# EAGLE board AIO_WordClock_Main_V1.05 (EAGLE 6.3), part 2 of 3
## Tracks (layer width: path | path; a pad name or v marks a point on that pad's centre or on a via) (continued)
+3V3  (via drill 0.5, 0.6) (continued)
  Bottom 0.406: 138.15,300.52 137.36,299.73 C104.1 136.66,299.65 C103.1 | 138.15,238.52 137.36,237.73 C204.1 136.66,237.66 C203.1 | 138.15,176.52 137.36,175.73 C304.1 136.66,175.66 C303.1 | 138.15,114.52 137.36,113.73 C404.1 136.66,113.66 C403.1 | 138.15,52.52 137.36,51.73 C504.1 136.66,51.66 C503.1 | U703.2 210.87,51.26 C704.1 208.22,51.26 208,51.47 208,55.03 | 198.96,55.03 208,55.03 | 208,55.03 211.05,58.08 242.42,58.08 v245.34,61 | C710.1 217.38,41.74 U704.45 220.44,41.74 v220.57,41.87 | C712.1 217.38,33.74 U704.35 220.47,33.74 v220.57,33.85 | C709.1 225.87,28.76 226.53,29.41 U704.25 226.53,31.68 v226.42,31.79 | C708.1 236.47,32.94 U704.15 233.36,32.94 v233.28,32.88 | C711.1 224.12,47.69 U704.53 224.12,44.49 v224.18,44.49 | C713.1 230.53,47.69 U704.61 230.53,44.62 v230.66,44.49 | R705.1 264.66,69.75 v264.52,69.89 | R706.1 R707.1 162.45,23.7 v163.43,24.68 | J701.4 227.56,331.51 309.22,331.51 311.13,329.6 311.13,85
  Bottom 0.61: v136.65,295.82 C103.1 | C203.1 136.66,234.26 v136.12,233.72 | C303.1 136.66,172.53 v135.87,171.74 | C403.1 136.66,110.56 v135.87,109.77 | C503.1 136.66,48.45 v135.87,47.66 | R701.1 196.67,96.33 198.99,94.02 198.96,55.03 198.96,53.13 198.96,51.09 198.96,49.06 | 236.42,30.82 v235.16,30.82 | 236.42,30.82 C714.1 | 236.42,30.82 236.58,30.67 v236.58,24.68 | v285.73,21.76 285.73,46.14 290.43,50.84 290.43,56.94 | 290.43,56.94 290.43,81.32 291.69,82.59 308.71,82.59 311.13,85 | R703.1 290.51,57.03 290.43,56.94 | v300.84,21.76 301.09,21.76 303.12,19.72 303.12,10.2 J701A.4
  Bottom 1.016: v131.04,295.82 v131.04,233.72 v131.04,171.74 v131.04,109.77 v131.04,47.66 v131.04,24.68 | v198.96,24.68 198.96,49.06 | v225.02,17.82 J702.3
+3V3A  (via drill 0.5)
  Top 0.406: J603.10 179.17,14.01 J603.9 177.65,16.8 162.79,16.8 161.9,15.91 161.9,10.94 v165.2,7.63 165.21,7.52 U602.4
  Bottom 0.406: C609.1 165.34,7.39 v165.2,7.63
D+
  Top 0.254: U602.15 171.71,11.94 172.57,11.09 178.54,11.09 179.05,10.58 179.05,9.56 179.17,9.44 J602.3
D-
  Top 0.254: U602.16 171.06,11.83 172.31,10.58 178.28,10.58 178.54,10.33 178.54,9.56 178.37,9.4 J602.2
DCF77#  (via drill 0.5, 0.6)
  Top 0.254: v255.5,23.03 v283.06,23.03 v294.87,23.03
  Bottom 0.254: v255.5,23.03 255.5,33.43 249.59,39.34 U704.7 | J701.2 228.19,329.73 228.83,330.37 308.97,330.37 310.11,329.22 310.11,86.53 307.95,84.37 290.81,84.37 288.65,82.21 288.65,51.73 283.69,46.78 283.69,24.8 283.06,24.17 v283.06,23.03 | v294.87,23.03 301.47,23.03 303.76,20.74 303.76,10.96 307.57,7.15 307.57,5.75 J701A.2
DISP-A0
  Bottom 0.254: J702.2 226.29,19.47 232.12,25.31 U704.18
DISP-CLK
  Bottom 0.254: J702.7 219.94,16.68 228.96,25.69 228.96,28.79 228.12,29.62 U704.23
DISP-CS#
  Bottom 0.254: J702.5 222.48,17.44 230.53,25.48 U704.20
DISP-DIN
  Bottom 0.254: J702.6 221.21,17.06 229.72,25.57 U704.21
DISP-RESET#
  Bottom 0.254: J702.4 223.75,17.82 231.32,25.39 U704.19
GND  (via drill 0.5, 3)
  Top 0.406: U601.HS 286.11,14.21 290.48,14.21 290.48,8.7 281.76,8.7 281.76,14.21 286.03,14.21 | U603.HS 236.58,14.21 240.92,14.21 240.92,8.73 232.23,8.73 232.23,14.19 236.53,14.19
  Bottom 0.254: U401.45 138.64,117.15 138.03,117.77
  Bottom 0.406: C710.2 217.38,40.94 U704.44 220.52,40.94 v220.57,40.88 | C712.2 217.38,32.94 U704.34 220.49,32.94 v220.57,32.86 | C709.2 227.32,28.61 U704.24 227.32,31.73 v227.38,31.79 | C708.2 236.47,33.74 U704.14 233.38,33.74 v233.28,33.85 | C711.2 223.32,47.69 U704.52 223.32,44.49 v223.17,44.49 | C713.2 229.72,47.69 U704.60 229.72,44.57 v229.64,44.49
  other vias: 219.81,49.82 230.74,53.89 226.04,53.46 210.67,53.38 226.93,38.14 164.57,33.36 177.65,33.36 177.52,72.73 164.57,72.73 164.44,95.21 177.65,95.21 164.57,134.71 177.52,134.71 177.65,157.19 164.44,157.19 164.44,219.17 177.4,196.81 177.65,219.17 164.57,196.81 164.57,258.79 177.52,258.79 164.44,281.27 177.65,281.27 164.57,320.89 177.52,320.89 143.49,302.1 143.49,240.12 143.49,178.02 143.49,116.04 143.49,54.07 240.39,18.38 246.1,11.39 248.51,8.22 240.39,4.66 252.58,18.25 252.58,10.12 266.42,19.65 269.98,12.79 274.04,10.76 276.45,11.39 283.57,1.31 282.3,18.38 246.74,6.31 274.55,8.22 286.11,11.47 236.58,11.47 233.15,13.43 233.15,12.16 233.15,10.89 233.15,9.62 234.29,13.43 234.29,12.16 234.29,10.89 234.29,9.62 240.01,9.62 238.86,9.62 238.86,10.89 240.01,10.89 240.01,12.16 238.86,12.16 238.86,13.43 240.01,13.43 282.68,13.43 282.68,12.16 282.68,10.89 282.68,9.62 283.82,13.43 283.82,12.16 283.82,10.89 283.82,9.62 288.52,13.43 288.52,12.16 288.52,10.89 288.52,9.62 289.66,13.43 289.66,12.16 289.66,10.89 289.66,9.62 276.33,1.31
  pour Bottom: 0,333.39 314,333.39 314,0.01 209.78,0.01 209.78,21.4 11.66,21.4 11.66,0.04 0,0.04 0,21.4
  pour Top: 0,333.39 314,333.39 314,0.01 209.78,0.01 209.78,21.4 11.66,21.4 11.66,0.04 0,0.04 0,21.4
GND1  (via drill 0.5)
  other vias: 46.46,16.8 45.95,11.17 43.23,7.79 58.65,11.98
  pour Bottom: 13.69,19.34 13.69,0.04 77.06,0.04 77.06,19.34
  pour Top: 13.69,19.34 13.69,0.04 77.06,0.04 77.06,19.34
GNDA  (via drill 0.5)
  other vias: 165.2,11.75 167.82,11.75 169.62,11.75 167.16,7.63
  pour Bottom: 158.98,19.47 158.98,0.04 207.75,0.04 207.75,19.47
  pour Top: 158.98,19.47 158.98,0.04 207.75,0.04 207.75,19.47
IR  (via drill 0.5)
  Top 0.254: U702.1 302.49,67.98 301.6,68.87 255.75,68.87 v247.88,61
  Bottom 0.254: U704.64 232.93,46.43 233.3,46.8 233.3,50.65 235.65,53 242.42,53 247.88,58.46 v247.88,61
KEY0
  Bottom 0.254: J702.8 218.67,16.3 222.53,20.15 U704.30
KEY1
  Bottom 0.254: J702.9 217.4,15.91 221.72,20.24 U704.31
KEY2
  Bottom 0.254: J702.10 216.13,15.53 220.93,20.33 U704.32
KEY3
  Bottom 0.254: J702.11 214.86,15.28 219.12,19.54 U704.33
LDR  (via drill 0.5, 0.6)
  Top 0.254: v264.52,67.86 257.28,67.86 v250.42,61 | v287.19,39.39 R708B.1
  Bottom 0.254: U704.63 232.12,46.44 232.59,46.9 232.59,50.68 235.39,53.48 242.14,53.48 247.12,58.46 247.12,61.38 247.75,62.02 249.4,62.02 v250.42,61 | v264.52,67.86 264.71,68.05 R705.2 C705.1 274.81,68.05 R708.1 275.46,39.41 R708B.1 | R708A.1 v287.19,39.39
LED0@U1  (via drill 0.5)
  Top 0.406: v140.44,309.03 138.79,307.38 23.98,307.38 18.52,312.84 18.52,313.73 D101.C
  Bottom 0.254: U101.2 141.25,306.87 140.44,307.69 v140.44,309.03
LED0@U2  (via drill 0.5)
  Top 0.406: v140.44,247.03 138.79,245.38 23.98,245.38 18.52,250.84 18.52,251.73 D201.C
  Bottom 0.254: U201.2 141.25,244.87 140.44,245.69 v140.44,247.03
LED0@U3  (via drill 0.5)
  Top 0.406: v140.44,185.03 138.79,183.38 23.98,183.38 18.52,188.84 18.52,189.73 D301.C
  Bottom 0.254: U301.2 141.25,182.87 140.44,183.69 v140.44,185.03
LED0@U4  (via drill 0.5)
  Top 0.406: v140.44,123.03 138.79,121.38 23.98,121.38 18.52,126.84 18.52,127.73 D401.C
  Bottom 0.254: U401.2 141.25,120.87 140.44,121.69 v140.44,123.03
LED0@U5  (via drill 0.5)
  Top 0.406: v140.44,61.03 138.79,59.38 23.98,59.38 18.52,64.84 18.52,65.73 D501.C
  Bottom 0.254: U501.2 141.25,58.87 140.44,59.68 v140.44,61.03
LED1@U1  (via drill 0.5)
  Top 0.406: v141.2,308.27 141.2,309.67 140.95,309.92 140.06,309.92 138.28,308.14 51.28,308.14 46.59,312.84 46.59,313.73 D102.C
  Bottom 0.254: U101.3 141.75,307.11 141.2,307.66 v141.2,308.27
LED1@U2  (via drill 0.5)
  Top 0.406: v141.2,246.27 141.2,247.67 140.95,247.92 140.06,247.92 138.28,246.14 51.28,246.14 46.59,250.84 46.59,251.74 D202.C
  Bottom 0.254: U201.3 141.75,245.11 141.2,245.66 v141.2,246.27
LED1@U3  (via drill 0.5)
  Top 0.406: v141.2,184.27 141.2,185.67 140.95,185.92 140.06,185.92 138.28,184.14 51.28,184.14 46.59,188.84 46.59,189.74 D302.C
  Bottom 0.254: U301.3 141.75,183.11 141.2,183.66 v141.2,184.27
LED1@U4  (via drill 0.5)
  Top 0.406: v141.2,122.27 141.2,123.67 140.95,123.92 140.06,123.92 138.28,122.14 51.28,122.14 46.59,126.84 46.59,127.73 D402.C
  Bottom 0.254: U401.3 141.75,121.11 141.2,121.66 v141.2,122.27
LED1@U5  (via drill 0.5)
  Top 0.406: v141.2,60.27 141.2,61.67 140.95,61.92 140.06,61.92 138.28,60.14 51.28,60.14 46.59,64.84 46.59,65.73 D502.C
  Bottom 0.254: U501.3 141.75,59.11 141.2,59.66 v141.2,60.27
LED2@U1  (via drill 0.5)
  Top 0.406: v141.96,309.03 141.96,310.05 141.33,310.68 139.55,310.68 137.77,308.9 78.59,308.9 74.78,312.71 74.78,313.67 D103.C
  Bottom 0.254: U101.4 142.25,307.35 141.96,307.63 v141.96,309.03
LED2@U2  (via drill 0.5)
  Top 0.406: v141.96,247.03 141.96,248.05 141.33,248.68 139.55,248.68 137.77,246.9 78.59,246.9 74.78,250.71 74.78,251.67 D203.C
  Bottom 0.254: U201.4 142.25,245.35 141.96,245.63 v141.96,247.03
LED2@U3  (via drill 0.5)
  Top 0.406: v141.96,185.03 141.96,186.05 141.33,186.68 139.55,186.68 137.77,184.9 78.59,184.9 74.78,188.71 74.78,189.67 D303.C
  Bottom 0.254: U301.4 142.25,183.35 141.96,183.63 v141.96,185.03
LED2@U4  (via drill 0.5)
  Top 0.406: v141.96,123.03 141.96,124.05 141.33,124.68 139.55,124.68 137.77,122.9 78.59,122.9 74.78,126.71 74.78,127.67 D403.C
  Bottom 0.254: U401.4 142.25,121.35 141.96,121.63 v141.96,123.03
LED2@U5  (via drill 0.5)
  Top 0.406: v141.96,61.03 141.96,62.05 141.33,62.68 139.55,62.68 137.77,60.9 78.59,60.9 74.78,64.71 74.78,65.67 D503.C
  Bottom 0.254: U501.4 142.25,59.35 141.96,59.63 v141.96,61.03
LED3@U1  (via drill 0.5)
  Top 0.406: v142.72,308.27 142.72,310.43 141.71,311.44 139.04,311.44 137.26,309.67 105.89,309.67 102.85,312.71 102.85,313.7 D104.C
  Bottom 0.254: U101.5 142.75,308.24 v142.72,308.27
LED3@U2  (via drill 0.5)
  Top 0.406: v142.72,246.27 142.72,248.43 141.71,249.44 139.04,249.44 137.26,247.67 105.89,247.67 102.85,250.71 102.85,251.7 D204.C
  Bottom 0.254: U201.5 142.75,246.24 v142.72,246.27
LED3@U3  (via drill 0.5)
  Top 0.406: v142.72,184.27 142.72,186.43 141.71,187.44 139.04,187.44 137.26,185.67 105.89,185.67 102.85,188.71 102.85,189.7 D304.C
  Bottom 0.254: U301.5 142.75,184.24 v142.72,184.27
LED3@U4  (via drill 0.5)
  Top 0.406: v142.72,122.27 142.72,124.43 141.71,125.44 139.04,125.44 137.26,123.67 105.89,123.67 102.85,126.71 102.85,127.7 D404.C
  Bottom 0.254: U401.5 142.75,122.24 v142.72,122.27
LED3@U5  (via drill 0.5)
  Top 0.406: v142.72,60.27 142.72,62.43 141.71,63.44 139.04,63.44 137.26,61.67 105.89,61.67 102.85,64.71 102.85,65.7 D504.C
  Bottom 0.254: U501.5 142.75,60.24 v142.72,60.27
LED4@U1  (via drill 0.5)
  Top 0.406: D105.C 141.18,313.75 144.25,310.68 v144.25,309.03
  Bottom 0.254: U101.8 v144.25,309.03
LED4@U2  (via drill 0.5)
  Top 0.406: D205.C 141.18,251.75 144.25,248.68 v144.25,247.03
  Bottom 0.254: U201.8 v144.25,247.03
LED4@U3  (via drill 0.5)
  Top 0.406: D305.C 141.18,189.75 144.25,186.68 v144.25,185.03
  Bottom 0.254: U301.8 v144.25,185.03
LED4@U4  (via drill 0.5)
  Top 0.406: D405.C 141.18,127.75 144.25,124.68 v144.25,123.03
  Bottom 0.254: U401.8 v144.25,123.03
LED4@U5  (via drill 0.5)
  Top 0.406: D505.C 141.18,65.75 144.25,62.68 v144.25,61.03
  Bottom 0.254: U501.8 v144.25,61.03
LED5@U1  (via drill 0.5)
  Top 0.406: v145.01,308.27 145.01,309.92 145.77,310.68 156.97,310.68 158.98,312.69 158.98,313.73 D106.C
  Bottom 0.254: U101.9 144.75,308.01 v145.01,308.27
LED5@U2  (via drill 0.5)
  Top 0.406: v145.01,246.27 145.01,247.92 145.77,248.68 156.97,248.68 158.98,250.69 158.98,251.73 D206.C
  Bottom 0.254: U201.9 144.75,246.01 v145.01,246.27
LED5@U3  (via drill 0.5)
  Top 0.406: v145.01,184.27 145.01,185.92 145.77,186.68 156.97,186.68 158.98,188.69 158.98,189.73 D306.C
  Bottom 0.254: U301.9 144.75,184.01 v145.01,184.27
LED5@U4  (via drill 0.5)
  Top 0.406: v145.01,122.27 145.01,123.92 145.77,124.68 156.97,124.68 158.98,126.69 158.98,127.73 D406.C
  Bottom 0.254: U401.9 144.75,122.01 v145.01,122.27
LED5@U5  (via drill 0.5)
  Top 0.406: v145.01,60.27 145.01,61.92 145.77,62.68 156.97,62.68 158.98,64.69 158.98,65.73 D506.C
  Bottom 0.254: U501.9 144.75,60.01 v145.01,60.27
LED6@U1  (via drill 0.5)
  Top 0.406: v145.77,309.03 146.66,309.92 184.3,309.92 187.1,312.71 D107.C
  Bottom 0.254: U101.10 145.25,307.44 145.77,307.96 v145.77,309.03
LED6@U2  (via drill 0.5)
  Top 0.406: v145.77,247.03 146.66,247.92 184.3,247.92 187.1,250.71 D207.C
  Bottom 0.254: U201.10 145.25,245.44 145.77,245.96 v145.77,247.03
LED6@U3  (via drill 0.5)
  Top 0.406: v145.77,185.03 146.66,185.92 184.3,185.92 187.1,188.71 D307.C
  Bottom 0.254: U301.10 145.25,183.44 145.77,183.96 v145.77,185.03
LED6@U4  (via drill 0.5)
  Top 0.406: v145.77,123.03 146.66,123.92 184.3,123.92 187.1,126.71 D407.C
  Bottom 0.254: U401.10 145.25,121.44 145.77,121.96 v145.77,123.03
LED6@U5  (via drill 0.5)
  Top 0.406: v145.77,61.03 146.66,61.92 184.3,61.92 187.1,64.71 D507.C
  Bottom 0.254: U501.10 145.25,59.44 145.77,59.96 v145.77,61.03
LED7@U1  (via drill 0.5)
  Top 0.406: v146.66,308.27 147.55,309.16 211.63,309.16 215.22,312.74 215.22,313.73 D108.C
  Bottom 0.254: U101.11 145.75,307.18 146.66,308.09 v146.66,308.27
LED7@U2  (via drill 0.5)
  Top 0.406: v146.66,246.27 147.55,247.16 211.63,247.16 215.22,250.74 215.22,251.73 D208.C
  Bottom 0.254: U201.11 145.75,245.18 146.66,246.09 v146.66,246.27
LED7@U3  (via drill 0.5)
  Top 0.406: v146.66,184.27 147.55,185.16 211.63,185.16 215.22,188.74 215.22,189.73 D308.C
  Bottom 0.254: U301.11 145.75,183.18 146.66,184.09 v146.66,184.27
LED7@U4  (via drill 0.5)
  Top 0.406: v146.66,122.27 147.55,123.16 211.63,123.16 215.22,126.74 215.22,127.73 D408.C
  Bottom 0.254: U401.11 145.75,121.18 146.66,122.09 v146.66,122.27
LED7@U5  (via drill 0.5)
  Top 0.406: v146.66,60.27 147.55,61.16 211.63,61.16 215.22,64.74 215.22,65.73 D508.C
  Bottom 0.254: U501.11 145.75,59.18 146.66,60.09 v146.66,60.27
LED8@U1  (via drill 0.5)
  Top 0.406: v150.6,303.19 155.81,308.4 238.99,308.4 243.31,312.71 D109.C
  Bottom 0.254: U101.17 149.04,302.65 149.58,303.19 v150.6,303.19
LED8@U2  (via drill 0.5)
  Top 0.406: v150.6,241.19 155.81,246.4 238.99,246.4 243.31,250.71 D209.C
  Bottom 0.254: U201.17 149.04,240.65 149.58,241.19 v150.6,241.19
LED8@U3  (via drill 0.5)
  Top 0.406: v150.6,179.19 155.81,184.4 238.99,184.4 243.31,188.71 D309.C
  Bottom 0.254: U301.17 149.04,178.65 149.58,179.19 v150.6,179.19
LED8@U4  (via drill 0.5)
  Top 0.406: v150.6,117.19 155.81,122.4 238.99,122.4 243.31,126.71 D409.C
  Bottom 0.254: U401.17 149.04,116.65 149.58,117.19 v150.6,117.19
LED8@U5  (via drill 0.5)
  Top 0.406: v150.6,55.19 155.81,60.4 238.99,60.4 243.31,64.71 D509.C
  Bottom 0.254: U501.17 149.04,54.65 149.58,55.19 v150.6,55.19
LED9@U1  (via drill 0.5)
  Top 0.406: v149.84,302.3 150.98,302.3 156.31,307.63 266.3,307.63 271.25,312.59 271.25,313.6 D110.C
  Bottom 0.254: U101.18 149.69,302.15 v149.84,302.3
LED9@U2  (via drill 0.5)
  Top 0.406: v149.84,240.3 150.98,240.3 156.31,245.63 266.3,245.63 271.25,250.59 271.25,251.6 D210.C
  Bottom 0.254: U201.18 149.69,240.15 v149.84,240.3
LED9@U3  (via drill 0.5)
  Top 0.406: v149.84,178.3 150.98,178.3 156.31,183.63 266.3,183.63 271.25,188.59 271.25,189.6 D310.C
  Bottom 0.254: U301.18 149.69,178.15 v149.84,178.3
LED9@U4  (via drill 0.5)
  Top 0.406: v149.84,116.3 150.98,116.3 156.31,121.63 266.3,121.63 271.25,126.59 271.25,127.6 D410.C
  Bottom 0.254: U401.18 149.69,116.15 v149.84,116.3
LED9@U5  (via drill 0.5)
  Top 0.406: v149.84,54.3 150.98,54.3 156.31,59.63 266.3,59.63 271.25,64.59 271.25,65.6 D510.C
  Bottom 0.254: U501.18 149.69,54.15 v149.84,54.3
LED10@U1  (via drill 0.5)
  Top 0.406: v150.6,301.41 151.36,301.41 156.82,306.87 293.6,306.87 299.44,312.71 299.44,313.69 D111.C
  Bottom 0.254: U101.19 149.5,301.65 149.73,301.41 v150.6,301.41
LED10@U2  (via drill 0.5)
  Top 0.406: v150.6,239.41 151.36,239.41 156.82,244.87 293.6,244.87 299.44,250.71 299.44,251.69 D211.C
  Bottom 0.254: U201.19 149.5,239.65 149.73,239.41 v150.6,239.41
LED10@U3  (via drill 0.5)
  Top 0.406: v150.6,177.41 151.36,177.41 156.82,182.87 293.6,182.87 299.44,188.71 299.44,189.69 D311.C
  Bottom 0.254: U301.19 149.5,177.65 149.73,177.41 v150.6,177.41
LED10@U4  (via drill 0.5)
  Top 0.406: v150.6,115.41 151.36,115.41 156.82,120.87 293.6,120.87 299.44,126.71 299.44,127.69 D411.C
  Bottom 0.254: U401.19 149.5,115.65 149.73,115.41 v150.6,115.41
LED10@U5  (via drill 0.5)
  Top 0.406: v150.6,53.41 151.36,53.41 156.82,58.87 293.6,58.87 299.44,64.71 299.44,65.69 D511.C
  Bottom 0.254: U501.19 149.5,53.65 149.73,53.41 v150.6,53.41
LED11@U1  (via drill 0.5)
  Top 0.406: D122.C 295.5,289.98 289.41,296.08 157.84,296.08 153.26,300.65 v149.84,300.65
  Bottom 0.254: U101.20 149.34,301.15 v149.84,300.65
LED11@U2  (via drill 0.5)
  Top 0.406: D222.C 295.5,227.98 289.41,234.08 160.91,234.08 156.34,238.65 v149.84,238.65
  Bottom 0.254: U201.20 149.34,239.15 v149.84,238.65
LED11@U3  (via drill 0.5)
  Top 0.406: D322.C 295.5,165.98 289.41,172.08 158.82,172.08 154.25,176.65 v149.84,176.65
  Bottom 0.254: U301.20 149.34,177.15 v149.84,176.65
LED11@U4  (via drill 0.5)
  Top 0.406: D422.C 295.5,103.98 289.41,110.08 160.7,110.08 156.13,114.65 v149.84,114.65
  Bottom 0.254: U401.20 149.34,115.15 v149.84,114.65
LED11@U5  (via drill 0.5)
  Top 0.406: D522.C 295.5,56.17 293.6,58.08 157.33,58.08 151.9,52.65 v149.84,52.65
  Bottom 0.254: U501.20 149.34,53.15 v149.84,52.65
LED12@U1  (via drill 0.5)
  Top 0.406: D121.C 267.44,289.09 267.44,289.6 261.72,295.31 146.79,295.31 v146.53,295.57
  Bottom 0.254: U101.26 145.75,296.61 146.53,295.82 v146.53,295.57
LED12@U2  (via drill 0.5)
  Top 0.406: D221.C 267.44,227.09 267.44,227.6 261.72,233.31 146.79,233.31 v146.53,233.57
  Bottom 0.254: U201.26 145.75,234.61 146.53,233.82 v146.53,233.57
LED12@U3  (via drill 0.5)
  Top 0.406: D321.C 267.44,165.09 267.44,165.6 261.72,171.31 146.79,171.31 v146.53,171.57
  Bottom 0.254: U301.26 145.75,172.61 146.53,171.82 v146.53,171.57
LED12@U4  (via drill 0.5)
  Top 0.406: D421.C 267.44,103.09 267.44,103.6 261.72,109.31 146.79,109.31 v146.53,109.57
  Bottom 0.254: U401.26 145.75,110.61 146.53,109.82 v146.53,109.57
LED12@U5  (via drill 0.5)
  Top 0.406: D521.C 267.44,41.09 267.44,54.65 264.77,57.32 157.84,57.32 155.55,55.03 155.55,48.94 153.93,47.31 146.79,47.31 v146.53,47.57
  Bottom 0.254: U501.26 145.75,48.61 146.53,47.82 v146.53,47.57
LED13@U1  (via drill 0.5)
  Top 0.406: v145.77,294.81 146.03,294.55 234.29,294.55 238.86,289.98 238.86,289.49 D120.C
  Bottom 0.254: U101.27 145.25,296.34 145.77,295.82 v145.77,294.81
LED13@U2  (via drill 0.5)
  Top 0.406: v145.77,232.81 146.03,232.55 234.29,232.55 238.86,227.98 238.86,227.49 D220.C
  Bottom 0.254: U201.27 145.25,234.34 145.77,233.82 v145.77,232.81
LED13@U3  (via drill 0.5)
  Top 0.406: v145.77,170.81 146.03,170.55 234.29,170.55 238.86,165.98 238.86,165.49 D320.C
  Bottom 0.254: U301.27 145.25,172.34 145.77,171.82 v145.77,170.81
LED13@U4  (via drill 0.5)
  Top 0.406: v145.77,108.81 146.03,108.55 234.29,108.55 238.86,103.98 238.86,103.49 D420.C
  Bottom 0.254: U401.27 145.25,110.34 145.77,109.82 v145.77,108.81
LED13@U5  (via drill 0.5)
  Top 0.406: v145.77,46.81 146.03,46.55 154.44,46.55 156.44,48.55 156.44,54.65 158.34,56.55 237.59,56.55 239.3,54.85 D520.C
  Bottom 0.254: U501.27 145.25,48.34 145.77,47.82 v145.77,46.81
LED14@U1  (via drill 0.5)
  Top 0.406: v145.01,295.57 145.01,294.3 145.52,293.79 207.11,293.79 211.18,289.73 211.18,289.07 D119.C
  Bottom 0.254: U101.28 144.75,295.83 v145.01,295.57
LED14@U2  (via drill 0.5)
  Top 0.406: v145.01,233.57 145.01,232.3 145.52,231.79 207.11,231.79 211.18,227.73 211.18,227.07 D219.C
  Bottom 0.254: U201.28 144.75,233.83 v145.01,233.57
LED14@U3  (via drill 0.5)
  Top 0.406: v145.01,171.57 145.01,170.3 145.52,169.79 207.11,169.79 211.18,165.73 211.18,165.07 D319.C
  Bottom 0.254: U301.28 144.75,171.83 v145.01,171.57
LED14@U4  (via drill 0.5)
  Top 0.406: v145.01,109.57 145.01,108.3 145.52,107.79 207.11,107.79 211.18,103.73 211.18,103.07 D419.C
  Bottom 0.254: U401.28 144.75,109.83 v145.01,109.57
LED14@U5  (via drill 0.5)
  Top 0.406: v145.01,47.57 145.01,46.3 145.52,45.79 207.11,45.79 211.18,41.73 211.18,41.07 D519.C
  Bottom 0.254: U501.28 144.75,47.83 v145.01,47.57
LED15@U1  (via drill 0.5)
  Top 0.406: D118.C 182.86,289.29 182.86,289.85 179.81,292.9 145.26,292.9 144.25,293.92 v144.25,294.8 v144.25,294.81
  Bottom 0.254: U101.29 v144.25,294.81
LED15@U2  (via drill 0.5)
  Top 0.406: D218.C 182.86,227.29 182.86,227.85 179.81,230.9 145.26,230.9 144.25,231.92 144.25,232.17 144.25,232.18 v144.25,232.81
  Bottom 0.254: U201.29 v144.25,232.81
LED15@U3  (via drill 0.5)
  Top 0.406: D318.C 182.86,165.29 182.86,165.85 179.81,168.9 145.26,168.9 144.25,169.92 v144.25,170.81
  Bottom 0.254: U301.29 v144.25,170.81
LED15@U4  (via drill 0.5)
  Top 0.406: v144.25,108.81 144.25,107.92 145.26,106.9 179.81,106.9 182.86,103.85 182.86,103.29 D418.C
  Bottom 0.254: U401.29 v144.25,108.81
LED15@U5  (via drill 0.5)
  Top 0.406: D518.C 182.86,41.29 182.86,41.85 179.81,44.9 145.26,44.9 144.25,45.92 v144.25,46.8 v144.25,46.81
  Bottom 0.254: U501.29 v144.25,46.81
LED16@U1  (via drill 0.5)
  Top 0.406: D117.C 154.92,289.13 154.92,289.73 152.5,292.14 144.76,292.14 142.75,294.15 142.75,295.54 v142.72,295.57
  Bottom 0.254: U101.32 142.75,295.59 v142.72,295.57
LED16@U2  (via drill 0.5)
  Top 0.406: v142.75,233.57 142.75,232.15 144.76,230.14 152.5,230.14 154.92,227.73 154.92,227.13 D217.C
  Bottom 0.254: U201.32 v142.75,233.57 142.72,233.57
LED16@U3  (via drill 0.5)
  Top 0.406: D317.C 154.92,165.13 154.92,165.73 152.5,168.14 144.76,168.14 142.75,170.15 142.75,171.54 v142.72,171.57
  Bottom 0.254: U301.32 142.75,171.59 v142.72,171.57
LED16@U4  (via drill 0.5)
  Top 0.406: v142.75,109.57 142.75,108.15 144.76,106.14 152.5,106.14 154.92,103.73 154.92,103.13 D417.C
  Bottom 0.254: U401.32 v142.75,109.57 142.72,109.57
LED16@U5  (via drill 0.5)
  Top 0.406: D517.C 154.92,41.13 154.92,41.73 152.5,44.14 144.76,44.14 142.75,46.15 142.75,47.54 v142.72,47.57
  Bottom 0.254: U501.32 142.75,47.59 v142.72,47.57
LED17@U1  (via drill 0.5)
  Top 0.406: 126.9,288.44 D116.C 127.48,289.63 127.48,290.36 130.15,293.03 141.07,293.03 141.96,293.92 v141.96,294.81
  Bottom 0.254: U101.33 142.25,296.11 141.96,295.82 v141.96,294.81
LED17@U2  (via drill 0.5)
  Top 0.406: 126.9,226.44 D216.C 127.48,227.63 127.48,228.36 130.15,231.03 141.07,231.03 141.96,231.92 v141.96,232.81
  Bottom 0.254: U201.33 142.25,234.11 141.96,233.82 v141.96,232.81
LED17@U3  (via drill 0.5)
  Top 0.406: 126.9,164.44 D316.C 127.48,165.63 127.48,166.36 130.15,169.03 141.07,169.03 141.96,169.92 v141.96,170.81
  Bottom 0.254: U301.33 142.25,172.11 141.96,171.82 v141.96,170.81
LED17@U4  (via drill 0.5)
  Top 0.406: 126.9,102.44 D416.C 127.48,103.63 127.48,104.36 130.15,107.03 141.07,107.03 141.96,107.92 v141.96,108.81
  Bottom 0.254: U401.33 142.25,110.11 141.96,109.82 v141.96,108.81
LED17@U5  (via drill 0.5)
  Top 0.406: 126.9,40.44 D516.C 127.48,41.63 127.48,42.36 130.15,45.03 141.07,45.03 141.96,45.92 v141.96,46.81
  Bottom 0.254: U501.33 142.25,48.11 141.96,47.82 v141.96,46.81
LED18@U1  (via drill 0.5)
  Top 0.406: v141.2,295.57 141.2,294.3 140.82,293.92 102.72,293.92 98.78,289.98 98.78,289.07 D115.C
  Bottom 0.254: U101.34 141.75,296.37 141.2,295.82 v141.2,295.57
LED18@U2  (via drill 0.5)
  Top 0.406: v141.2,233.57 141.2,232.3 140.82,231.92 102.72,231.92 98.78,227.98 98.78,227.07 D215.C
  Bottom 0.254: U201.34 141.75,234.37 141.2,233.82 v141.2,233.57
LED18@U3  (via drill 0.5)
  Top 0.406: v141.2,171.57 141.2,170.3 140.82,169.92 102.72,169.92 98.78,165.98 98.78,165.07 D315.C
  Bottom 0.254: U301.34 141.75,172.37 141.2,171.82 v141.2,171.57
LED18@U4  (via drill 0.5)
  Top 0.406: v141.2,109.57 141.2,108.3 140.82,107.92 102.72,107.92 98.78,103.98 98.78,103.07 D415.C
  Bottom 0.254: U401.34 141.75,110.37 141.2,109.82 v141.2,109.57
LED18@U5  (via drill 0.5)
  Top 0.406: v141.2,47.57 141.2,46.3 140.82,45.92 102.72,45.92 98.78,41.98 98.78,41.07 D515.C
  Bottom 0.254: U501.34 141.75,48.37 141.2,47.82 v141.2,47.57
LED19@U1  (via drill 0.5)
  Top 0.406: v140.44,294.81 75.54,294.81 70.84,290.11 70.84,289.19 D114.C
  Bottom 0.254: U101.35 141.25,296.63 140.44,295.82 v140.44,294.81
LED19@U2  (via drill 0.5)
  Top 0.406: v140.44,232.81 75.54,232.81 70.84,228.11 70.84,227.19 D214.C
  Bottom 0.254: U201.35 141.25,234.64 140.44,233.82 v140.44,232.81
LED19@U3  (via drill 0.5)
  Top 0.406: v140.44,170.81 75.54,170.81 70.84,166.11 70.84,165.19 D314.C
  Bottom 0.254: U301.35 141.25,172.64 140.44,171.82 v140.44,170.81
LED19@U4  (via drill 0.5)
  Top 0.406: v140.44,108.81 75.54,108.81 70.84,104.11 70.84,103.19 D414.C
  Bottom 0.254: U401.35 141.25,110.63 140.44,109.82 v140.44,108.81
LED19@U5  (via drill 0.5)
  Top 0.406: v140.44,46.81 75.54,46.81 70.84,42.11 70.84,41.19 D514.C
  Bottom 0.254: U501.35 141.25,48.63 140.44,47.82 v140.44,46.81
LED20@U1  (via drill 0.5)
  Top 0.406: v137.14,301.16 53.7,301.16 42.77,290.23 42.77,289.22 D113.C
  Bottom 0.254: U101.41 v137.14,301.15 v137.14,301.16
LED20@U2  (via drill 0.5)
  Top 0.406: v137.14,239.16 53.7,239.16 42.77,228.24 42.77,227.22 D213.C
  Bottom 0.254: U201.41 v137.14,239.15 v137.14,239.16
LED20@U3  (via drill 0.5)
  Top 0.406: v137.14,177.16 53.7,177.16 42.77,166.24 42.77,165.22 D313.C
  Bottom 0.254: U301.41 v137.14,177.15 v137.14,177.16
LED20@U4  (via drill 0.5)
  Top 0.406: v137.14,115.16 53.7,115.16 42.77,104.23 42.77,103.22 D413.C
  Bottom 0.254: U401.41 v137.14,115.15 v137.14,115.16
LED20@U5  (via drill 0.5)
  Top 0.406: v137.14,53.16 53.7,53.16 42.77,42.23 42.77,41.22 D513.C
  Bottom 0.254: U501.41 v137.14,53.15 v137.14,53.16
LED21@U1  (via drill 0.5)
  Top 0.406: D112.C 14.56,289.11 14.56,297.2 23.98,306.62 131.8,306.62 v136.5,301.92
  Bottom 0.254: U101.42 137.79,301.65 137.52,301.92 v136.5,301.92
LED21@U2  (via drill 0.5)
  Top 0.406: v136.5,239.92 26.38,239.92 14.56,228.11 14.56,227.12 D212.C
  Bottom 0.254: U201.42 137.79,239.65 137.52,239.92 v136.5,239.92
LED21@U3  (via drill 0.5)
  Top 0.406: v136.5,177.92 131.79,182.62 23.94,182.62 14.5,173.19 D312.C 14.56,165.12
  Bottom 0.254: U301.42 137.79,177.65 137.52,177.92 v136.5,177.92
LED21@U4  (via drill 0.5)
  Top 0.406: v136.5,115.92 26.38,115.92 14.56,104.11 14.56,103.12 D412.C
  Bottom 0.254: U401.42 137.79,115.65 137.52,115.92 v136.5,115.92
LED21@U5  (via drill 0.5)
  Top 0.406: v136.5,53.92 v136.5,53.91 131.87,58.54 24.21,58.54 14.56,48.89 14.56,41.11 D512.C
  Bottom 0.254: U501.42 137.79,53.65 137.52,53.92 v136.5,53.92
MATRIX-OE#  (via drill 0.5)
  Top 0.254: v159.62,48.3 225.4,48.3 v225.78,47.92
  Bottom 0.254: U101.24 148.92,299.15 151.61,296.46 151.61,237.15 | 151.61,175.15 151.61,237.15 | 151.61,175.15 151.61,113.17 | U401.24 151.59,113.15 151.61,113.17 | U301.24 151.61,175.15 | U201.24 151.61,237.15 | 151.61,113.17 151.61,51.17 | 151.61,51.17 151.61,50.59 153.9,48.3 v159.62,48.3 | U501.24 151.59,51.15 151.61,51.17 | U704.55 225.72,47.86 v225.78,47.92
MATRIX-PWR  (via drill 0.5)
  Top 0.254: v276.07,12.74 U601.3 | v254.74,22.26 v276.07,22.26
  Bottom 0.254: v276.07,22.26 v276.07,12.74 | v254.74,22.26 253.98,23.03 253.98,32.54 248.77,37.74 U704.9
MATRIX-SCL  (via drill 0.5)
  Top 0.254: v233.17,23.41 232.79,23.79 158.6,23.79 v158.34,23.54
  Bottom 0.254: R113.1 158.98,297.22 160.63,295.57 160.63,235.24 | 160.63,173.52 160.63,235.24 | 160.63,173.52 160.63,111.55 | 160.63,111.55 160.63,49.57 | 160.63,235.24 R213.1 | R313.1 160.63,173.52 | 160.63,111.55 R413.1 | 160.63,49.57 R513.1 | v233.17,23.41 R710.1 | 160.63,49.57 160.63,27.98 160.15,27.5 R706.2 158.34,23.6 v158.34,23.54
MATRIX-SDA  (via drill 0.5)
  Top 0.254: v161.77,237.28 v159.74,237.28 | v159.79,175.53 v161.77,175.53 | v161.77,113.58 v159.87,113.58 | v161.77,51.6 v158.85,51.6 | v235.21,23.41 234.29,23.41 233.6,22.72 232.69,22.72 232.06,23.36 164.75,23.36 v164.44,23.05
  Bottom 0.254: R112.1 158.37,299.23 161.9,295.7 v161.77,237.28 v161.77,175.53 v161.77,113.58 v161.77,51.6 161.77,27.98 162.18,27.57 R707.2 162.19,25.39 163.73,25.39 164.44,24.68 v164.44,23.05 | v159.74,237.28 R212.1 | R312.1 v159.79,175.53 | v159.87,113.58 R412.1 | v235.21,23.41 R709.1 | v158.85,51.6 R512.1
N$1
  Bottom 0.254: U704.16 234.47,32.14 234.47,30.52 235.21,29.78 R709.2
N$2
  Bottom 0.254: U704.17 232.93,26.54 R710.2
N$3
  Top 0.406: U603.3 246.86,10.2 247.88,9.18 250.67,9.18 251.4,8.46 R611.1 252.2,8.17 252.58,7.79 252.58,4.48 252.2,4.1 R608.2
N$4
  Top 0.406: U603.6 249.44,14.01 R610.2 | R610.2 C605.2 | R610.2 R609.2 R612.1
N$5
  Top 0.406: R603.2 274.73,2.89 274.17,2.33 271.5,2.33 | R603.3 271.5,1.89 271.5,2.33 | U601.6 275.82,8.93 275.06,9.69 271.16,9.69 | C601.2 271.12,8.71 | C601.2 271.16,9.69 | 271.16,9.69 R604.1 | 271.5,2.33 269.85,2.33 269.34,2.83 269.34,8.17 269.85,8.68 C601.2
N$6
  Top 0.406: U601.5 276.07,10.2 273.53,12.74 C603.1
N$7
  Top 0.406: U601.2 272.43,14.01 R601.2
N$8
  Top 0.406: C612.1 248.51,10.2 245.97,12.74 U603.5
N$9  (via drill 0.5)
  Top 0.254: v236.32,49.44 231.07,49.44 226.53,44.89 v226.53,43.68
  Bottom 0.254: J703.1 257.66,20.87 257.66,41.64 249.86,49.44 v236.32,49.44 | v226.53,43.68 U704.56
N$10
  Top 0.406: R607.2 251.4,6.43 250.67,7.15 247.88,7.15 246.1,8.93 U603.2
N$11  (via drill 0.5, 0.6)
  Top 0.254: v235.56,48.68 231.39,48.68 227.32,44.69 v227.32,44.44 | v251.06,24.8 v256.77,24.8
  Bottom 0.254: v235.56,48.68 249.57,48.68 256.9,41.35 256.9,24.8 | 256.9,24.8 J703.5 | U703.1 213.02,51.05 214.61,52.64 214.8,52.64 R704.2 219.16,48.91 226.06,48.91 226.87,48.1 226.87,46.88 227.32,46.43 U704.57 v227.32,44.44 | J704.6 249.78,25.44 250.42,24.8 v251.06,24.8 | v256.77,24.8 256.9,24.8
N$12
  Bottom 0.254: C707.1 230.34,50.61 XTAL701.3 228.3,50.48 228.3,47.05 228.93,46.43 U704.59
N$13
  Bottom 0.254: C706.1 220.21,53.11 XTAL701.1 222.25,53.11 222.84,52.52 225,52.52 226.67,50.84 226.67,49.44 227.56,48.55 227.56,47.03 228.12,46.47 U704.58
N$14  (via drill 0.5)
  Top 0.254: U602.17 170.41,12.58 170.64,12.36 170.64,11.44 v170.54,11.32
  Bottom 0.254: v170.54,11.32 170.46,11.39 170.46,13.03 C610.1
N$15  (via drill 0.5)
  Top 0.406: L601.2 v168.25,15.28 168.46,15.07 U602.20
  Bottom 0.254: C608.1 166.92,12.01 165.58,10.68 165.58,10.52 R606.1
  Bottom 0.406: 167.24,15.28 166.86,15.28 C607.1 | 167.24,15.28 v168.25,15.28 | C608.1 166.92,14.96 167.24,15.28
N$16
  Top 0.406: XTAL801.2 39.22,5.88 U801.5
N$19
  Top 0.406: X503.1 D523.C
N$20
  Top 0.406: XTAL801.1 38.71,4.61 U801.6
N$21
  Top 0.406: U801.13 53.19,7.15 XTAL802.2
N$22
  Top 0.406: U801.14 52.94,8.42 XTAL802.1
N$23
  Top 0.254: C805.1 38.16,10.96
  Top 0.406: 38.16,10.96 U801.1 42.01,10.96 42.39,11.34 | C805.1 C804.1 33.67,11.05 X801.1 | 42.39,11.34 C806.1 44.14,13.62 C807.1 44.78,14.26 44.93,14.26 45.99,15.32 R802.1 | U801.12 47.85,5.88 42.39,11.34
N$24
  Top 0.406: R802.2 48.23,13.62 C808.1 52.8,13.88 J801.4 52.94,17.18 53.57,17.82 59.32,17.82 R801.1
N$25
  Top 0.406: U801.7 38.81,3.34 38.41,2.94 38.09,2.94 C801.1
N$26
  Top 0.406: C802.1 54.29,0.93 49,0.93 47.85,2.07 U801.8 C801.2
N$27
  Top 0.406: U801.9 C802.2
N$28
  Top 0.406: U801.10 54.17,3.34 C803.1
N$29
  Top 0.406: U801.11 C803.2
N$30  (via drill 0.5)
  Top 0.406: v49,9.69 U801.15
  Bottom 0.406: J801.3 54.2,12.99 53.44,12.23 49.25,12.23 48.62,11.6 48.62,10.07 v49,9.69
N$31
  Top 0.406: U801.2 38.42,9.69 C805.2 C804.2 32.02,9.35 X802.1
N$32
  Top 0.406: J801.2 56.49,12.99 61.32,12.99 Q801.3 61.32,13.73 61.75,14.16 61.75,16.26 R801.2
N$33
  Top 0.406: R803.2 59.94,10.96 Q801.1
N$34
  Top 0.406: U801.16 R803.1
N$36
  Bottom 0.406: R701.2 194.96,101.55 194.84,101.44 | 194.84,101.44 C701.1 | 194.84,101.44 193.22,101.44 U701.1
N$38  (via drill 0.5)
  Top 0.406: v136.88,78.14 137.77,79.03 138.41,79.03 138.53,78.91 309.48,78.91 312.01,76.37 312.01,25.44 J501.2 309.86,21.25 309.86,15.41 J501A.2
  Bottom 0.254: U501.43 138.02,54.15 137.21,54.95
  Bottom 0.406: 137.21,54.95 137.21,77.31 136.88,77.64 v136.88,78.14
N$39
  Bottom 0.61: R703.2 303.9,58.72 C703.1 U702.2
N$40  (via drill 0.5)
  Top 0.406: v150.61,13.2 D523.A
  Bottom 0.406: R525.2 150.61,6.24 v150.61,13.2
N$41  (via drill 0.5)
  Top 0.406: v138.03,78.14 309.09,78.14 311.13,76.11 311.13,27.09 J501.4
  Bottom 0.254: U501.44 138.41,54.65 138.03,55.03
  Bottom 0.406: v138.03,78.14 138.03,55.03 | J501.4 310.11,23.54 310.11,13.12 J501A.4
N$42
  Bottom 0.406: R525.1 150.61,4.54 X501.1
N$44
  Bottom 0.406: R526.1 X502.1
N$45  (via drill 0.5)
  Top 0.406: v134.61,6.2 v134.6,6.2 D524.C
  Bottom 0.406: v134.61,6.2 X504.1
N$46  (via drill 0.5)
  Top 0.406: v130.61,6.3 v130.6,6.3 D524.A
  Bottom 0.406: v130.61,6.3 R526.2
N$47
  pour Top: 138.91,19.4 138.91,0 156.91,0 156.91,19.4
  pour Top: 118.91,19.4 118.91,0 136.91,0 136.91,19.4
  pour Top: 98.91,19.4 98.91,0 116.91,0 116.91,19.4
  pour Top: 78.91,19.4 78.91,0 96.91,0 96.91,19.4
  pour Bottom: 78.91,19.4 78.91,0 96.91,0 96.91,19.4
  pour Bottom: 98.91,19.4 98.91,0 116.91,0 116.91,19.4
  pour Bottom: 118.91,19.4 118.91,0 136.91,0 136.91,19.4
  pour Bottom: 138.91,19.4 138.91,0 156.91,0 156.91,19.4
N$48  (via drill 0.5)
  Top 0.406: v137.14,116.75 16.61,116.75 6.58,106.72 6.58,27.6 8.87,25.31 8.87,23.28 J401.2 8.87,21.25 8.87,14.77 J401A.2
  Bottom 0.254: U401.43 138.12,116.15 137.52,116.75 v137.14,116.75
N$54  (via drill 0.5)
  Top 0.406: v136.5,117.64 15.98,117.51 5.56,107.1 5.56,27.09 J401.4 4.8,24.8 4.04,24.04 4.04,11.85 4.67,11.22 J401A.4
  Bottom 0.254: U401.44 138.51,116.65 137.52,117.64 v136.5,117.64
N$55
  Top 0.406: X403.1 D423.C
N$56  (via drill 0.5)
  Top 0.406: v101.31,13.2 D423.A
  Bottom 0.406: R425.2 v101.31,13.2
N$57
  Bottom 0.406: X401.1 R425.1
N$58
  Bottom 0.406: R426.1 X402.1
N$60  (via drill 0.5)
  Top 0.406: D424.C v85.21,6.2
  Bottom 0.406: v85.21,6.2 X404.1
N$62  (via drill 0.5)
  Top 0.406: v81.21,6.2 D424.A
  Bottom 0.406: v81.21,6.2 R426.2
N$69
  Top 1.016: J603.2 188.06,14.01 | 188.06,14.01 J603.1 189.84,15.79 196.22,15.79 J601.1 | 188.06,14.01 J603.3
N$70  (via drill 0.5)
  Top 0.254: v163.93,2.83 163.26,3.5 U602.1
  Bottom 0.254: J603.5 184.25,4.1 182.98,2.83 v163.93,2.83
N$71  (via drill 0.5)
  Top 0.254: v166.47,3.6 165.86,4.2 U602.5
  Bottom 0.254: J603.7 181.71,10.2 183.49,8.42 183.49,4.36 182.73,3.6 v166.47,3.6
N$73
  Top 0.406: R602.2 271.16,4.63 R603.1
N$87  (via drill 0.5)
  Top 0.406: L601.1 173.2,15.28 | 173.2,15.28 C606.1 | 173.2,15.28 v173.2,14.14 | J602.1 177.57,6.44 178.16,5.86 v178.54,5.86
  Bottom 0.406: v173.2,14.14 178.16,14.14 179.17,13.12 179.17,11.98 179.94,11.22 179.94,6.24 179.55,5.86 v178.54,5.86
N$88  (via drill 0.5)
  Top 0.254: U602.19 169.11,12.46 168.76,12.1 v168.76,11.32
  Bottom 0.254: v168.76,11.32 168.76,10.24 R605.2 R606.2
PA3
  Bottom 0.254: U704.1 243.72,44.14 245.97,46.39 X9.P$1
PA4
  Bottom 0.254: U704.2 244.19,43.34 245.97,45.12 X10.P$1
PA5
  Bottom 0.254: U704.3 244.66,42.54 245.97,43.85 X11.P$1
PA6
  Bottom 0.254: U704.4 245.76,41.74 246.61,42.58 X12.P$1
PA7
  Bottom 0.254: U704.5 246.87,40.94 X13.P$1
PB0
  Bottom 0.254: U704.6 248.61,40.14 X14.P$1
PB4  (via drill 0.6)
  Top 0.254: X15.P$1 249.15,36.23 249.78,35.6 v249.78,33.7
  Bottom 0.254: U704.10 245.91,36.94 X15.P$1 | v249.78,33.7 J704.5
PB5
  Bottom 0.254: U704.11 235.21,36.14 235.43,36.36 243.82,36.36 245.21,34.96 X16.P$1 249.78,34.96 252.32,32.42 J704.9
PB6  (via drill 0.6)
  Top 0.254: X17.P$1 246.61,32.42 v245.34,31.16
  Bottom 0.254: U704.12 235.22,35.34 235.61,35.73 243.31,35.73 245.34,33.7 X17.P$1 | v245.34,31.16 245.34,30.52 245.78,30.08 J704.1
PB7
  Bottom 0.254: U704.13 235.21,34.54 235.84,35.17 242.85,35.17 245.59,32.42 X18.P$1 J704.3
PE0
  Bottom 0.254: U704.36 218.64,34.54 218.03,35.14 206.66,35.14 204.57,33.06 X1.P$1
PE1
  Bottom 0.254: X2.P$1 204.7,34.33 206.13,35.76 218.2,35.76 218.62,35.34 U704.37
PE2
  Bottom 0.254: U704.38 218.69,36.14 218.52,36.31 204.78,36.31 X3.P$1
PE3
  Bottom 0.254: U704.39 201.59,36.94 X4.P$1
PE4
  Bottom 0.254: U704.40 204.47,37.74 X5.P$1
PE5
  Bottom 0.254: X6.P$1 204.45,39.41 205.53,38.33 218.43,38.33 218.64,38.54 U704.41
PE6
  Bottom 0.254: U704.42 218.62,39.34 218.21,38.93 206.07,38.93 204.32,40.68 X7.P$1
PE7
  Bottom 0.254: U704.43 218.64,40.14 218.06,39.56 206.83,39.56 204.45,41.95 X8.P$1
PIR  (via drill 0.5)
  Top 0.254: v195.68,55.64 v231.9,55.64
  Bottom 0.254: v195.68,55.64 195.68,88.81 189.71,94.78 U701.2 | U704.62 231.32,46.45 231.9,47.03 v231.9,55.64
  Bottom 0.406: C702.1 U701.2 R702.1 191.28,99.95 190.98,100.24
R1@U1
  Top 0.406: R101.2 15.65,321.2 D101.A
R1@U2
  Top 0.406: R201.2 15.65,259.2 D201.A
R1@U3
  Top 0.406: R301.2 15.65,197.2 D301.A
R1@U4
  Top 0.406: R401.2 15.65,135.2 D401.A
R1@U5
  Top 0.406: R501.2 15.65,73.2 D501.A
R2@U1
  Top 0.406: R102.2 43.75,321.2 D102.A
R2@U2
  Top 0.406: R202.2 43.75,259.2 D202.A
R2@U3
  Top 0.406: R302.2 43.75,197.2 D302.A
R2@U4
  Top 0.406: R402.2 43.75,135.2 D402.A
R2@U5
  Top 0.406: R502.2 43.75,73.2 D502.A
R3@U1
  Top 0.406: R103.2 71.85,321.2 D103.A
R3@U2
  Top 0.406: R203.2 71.85,259.2 D203.A
R3@U3
  Top 0.406: R303.2 71.85,197.2 D303.A
R3@U4
  Top 0.406: R403.2 71.85,135.2 D403.A
R3@U5
  Top 0.406: R503.2 71.85,73.2 D503.A
R4@U1
  Top 0.406: R104.2 99.95,321.2 D104.A
R4@U2
  Top 0.406: R204.2 99.95,259.2 D204.A
R4@U3
  Top 0.406: R304.2 99.95,197.2 D304.A
R4@U4
  Top 0.406: R404.2 99.95,135.2 D404.A
R4@U5
  Top 0.406: R504.2 99.95,73.2 D504.A
R5@U1
  Top 0.406: R105.2 128.05,321.2 D105.A
R5@U2
  Top 0.406: R205.2 128.05,259.2 D205.A
R5@U3
  Top 0.406: R305.2 128.05,197.2 D305.A
R5@U4
  Top 0.406: R405.2 128.05,135.2 D405.A
R5@U5
  Top 0.406: R505.2 128.05,73.2 D505.A
R6@U1
  Top 0.406: R106.2 156.15,321.2 D106.A
R6@U2
  Top 0.406: R206.2 156.15,259.2 D206.A
R6@U3
  Top 0.406: R306.2 156.15,197.2 D306.A
R6@U4
  Top 0.406: R406.2 156.15,135.2 D406.A
R6@U5
  Top 0.406: R506.2 156.15,73.2 D506.A
R7@U1
  Top 0.406: R107.2 184.25,321.2 D107.A
R7@U2
  Top 0.406: R207.2 184.25,259.2 D207.A
R7@U3
  Top 0.406: R307.2 184.25,197.2 D307.A
R7@U4
  Top 0.406: R407.2 184.25,135.2 D407.A
R7@U5
  Top 0.406: R507.2 184.25,73.2 D507.A
R8@U1
  Top 0.406: R108.2 212.35,321.2 D108.A
R8@U2
  Top 0.406: R208.2 212.35,259.2 D208.A
R8@U3
  Top 0.406: R308.2 212.35,197.2 D308.A
R8@U4
  Top 0.406: R408.2 212.35,135.2 D408.A
R8@U5
  Top 0.406: R508.2 212.35,73.2 D508.A
R9@U1
  Top 0.406: R109.2 240.45,321.2 D109.A
R9@U2
  Top 0.406: R209.2 240.45,259.2 D209.A
R9@U3
  Top 0.406: R309.2 240.45,197.2 D309.A
R9@U4
  Top 0.406: R409.2 240.45,135.2 D409.A
R9@U5
  Top 0.406: R509.2 240.45,73.2 D509.A
R10@U1
  Top 0.406: R110.2 268.55,321.2 D110.A
R10@U2
  Top 0.406: R210.2 268.55,259.2 D210.A
R10@U3
  Top 0.406: R310.2 268.55,197.2 D310.A
R10@U4
  Top 0.406: R410.2 268.55,135.2 D410.A
R10@U5
  Top 0.406: R510.2 268.55,73.2 D510.A
R11@U1
  Top 0.406: R111.2 296.65,321.2 D111.A
R11@U2
  Top 0.406: R211.2 296.65,259.2 D211.A
R11@U3
  Top 0.406: R311.2 296.65,197.2 D311.A
R11@U4
  Top 0.406: R411.2 296.65,135.2 D411.A
R11@U5
  Top 0.406: R511.2 296.65,73.2 D511.A
R12@U1
  Top 0.406: R114.1 17.35,281.6 D112.A
R12@U2
  Top 0.406: R214.1 17.35,219.6 D212.A
R12@U3
  Top 0.406: R314.1 17.35,157.6 D312.A
R12@U4
  Top 0.406: R414.1 17.35,95.6 D412.A
R12@U5
  Top 0.406: R514.1 17.35,33.6 D512.A
R13@U1
  Top 0.406: R115.1 45.45,281.6 D113.A
R13@U2
  Top 0.406: R215.1 45.45,219.6 D213.A
R13@U3
  Top 0.406: R315.1 45.45,157.6 D313.A
R13@U4
  Top 0.406: R415.1 45.45,95.6 D413.A
R13@U5
  Top 0.406: R515.1 45.45,33.6 D513.A
R14@U1
  Top 0.406: R116.1 73.55,281.6 D114.A
R14@U2
  Top 0.406: R216.1 73.55,219.6 D214.A
R14@U3
  Top 0.406: R316.1 73.55,157.6 D314.A
R14@U4
  Top 0.406: R416.1 73.55,95.6 D414.A
R14@U5
  Top 0.406: R516.1 73.55,33.6 D514.A
R15@U1
  Top 0.406: R117.1 101.65,281.6 D115.A
R15@U2
  Top 0.406: R217.1 101.65,219.6 D215.A
R15@U3
  Top 0.406: R317.1 101.65,157.6 D315.A
R15@U4
  Top 0.406: R417.1 101.65,95.6 D415.A
R15@U5
  Top 0.406: R517.1 101.65,33.6 D515.A
R16@U1
  Top 0.406: R118.1 129.75,282.75 D116.A
R16@U2
  Top 0.406: R218.1 129.75,220.75 D216.A
R16@U3
  Top 0.406: R318.1 129.75,158.75 D316.A
R16@U4
  Top 0.406: R418.1 129.75,96.75 D416.A
R16@U5
  Top 0.406: R518.1 129.75,34.75 D516.A
R17@U1
  Top 0.406: R119.1 157.85,282.75 D117.A
R17@U2
  Top 0.406: R219.1 157.85,220.75 D217.A
R17@U3
  Top 0.406: R319.1 157.85,158.75 D317.A
R17@U4
  Top 0.406: R419.1 157.85,96.75 D417.A
R17@U5
  Top 0.406: R519.1 157.85,34.75 D517.A
R18@U1
  Top 0.406: R120.1 185.95,282.75 D118.A
R18@U2
  Top 0.406: R220.1 185.95,220.75 D218.A
R18@U3
  Top 0.406: R320.1 185.95,158.75 D318.A
R18@U4
  Top 0.406: R420.1 185.95,96.75 D418.A
R18@U5
  Top 0.406: R520.1 185.95,34.75 D518.A
R19@U1
  Top 0.406: R121.1 214.05,282.75 D119.A
R19@U2
  Top 0.406: R221.1 214.05,220.75 D219.A
R19@U3
  Top 0.406: R321.1 214.05,158.75 D319.A
R19@U4
  Top 0.406: R421.1 214.05,96.75 D419.A
R19@U5
  Top 0.406: R521.1 214.05,34.75 D519.A
R20@U1
  Top 0.406: R122.1 242.15,282.75 D120.A
R20@U2
  Top 0.406: R222.1 242.15,220.75 D220.A
R20@U3
  Top 0.406: R322.1 242.15,158.75 D320.A
R20@U4
  Top 0.406: R422.1 242.15,96.75 D420.A
R20@U5
  Top 0.406: R522.1 242.15,34.75 D520.A
R21@U1
  Top 0.406: R123.1 270.25,282.75 D121.A
R21@U2
  Top 0.406: R223.1 270.25,220.75 D221.A
R21@U3
  Top 0.406: R323.1 270.25,158.75 D321.A
R21@U4
  Top 0.406: R423.1 270.25,96.75 D421.A
R21@U5
  Top 0.406: R523.1 270.25,34.75 D521.A
R22@U1
  Top 0.406: R124.1 298.35,282.75 D122.A
R22@U2
  Top 0.406: R224.1 298.35,220.75 D222.A
R22@U3
  Top 0.406: R324.1 298.35,158.75 D322.A
R22@U4
  Top 0.406: R424.1 298.35,96.75 D422.A
R22@U5
  Top 0.406: R524.1 298.35,34.75 D522.A
RCV-EN#  (via drill 0.5, 0.6)
  Top 0.254: v254.74,23.79 v284.2,23.79 v296.14,23.79
  Bottom 0.254: v254.74,23.79 254.74,33.03 249.23,38.54 U704.8 | J701.3 226.93,329.99 227.81,330.88 309.09,330.88 310.62,329.35 310.62,86.4 308.08,83.86 291.06,83.86 289.15,81.95 289.15,51.47 284.2,46.52 v284.2,23.79 | v296.14,23.79 301.6,23.79 304.39,20.99 304.39,11.22 308.84,6.77 J701A.3
RXD  (via drill 0.5)
  Top 0.254: v237.09,50.2 230.79,50.2 226.43,45.84 v220.01,45.84
  Bottom 0.254: J604.7 258.8,9.06 263.12,13.37 263.12,17.06 258.42,21.76 258.42,41.93 250.14,50.2 v237.09,50.2 | v220.01,45.84 220.82,45.84 U704.49
SCL@U1  (via drill 0.5)
  Top 0.254: v140.74,299.38 144.76,299.38 145.9,298.24 151.49,298.24 v151.74,297.98
  Bottom 0.254: U101.38 140.47,299.65 v140.74,299.38 | v151.74,297.98 152.5,297.22 R113.2
SCL@U2  (via drill 0.5)
  Top 0.254: v140.74,237.28 144.76,237.28 145.65,236.39 153.26,236.39 v154.41,235.24
  Bottom 0.254: U201.38 140.37,237.65 v140.74,237.28 | v154.41,235.24 R213.2
SCL@U3  (via drill 0.5)
  Top 0.254: v140.74,175.17 144.88,175.17 145.75,174.31 153.49,174.31 v154.28,173.52
  Bottom 0.254: U301.38 140.27,175.65 v140.74,175.17 | v154.28,173.52 R313.2
SCL@U4  (via drill 0.5)
  Top 0.254: v140.74,113.32 144.63,113.32 145.52,112.44 153.52,112.44 v154.41,111.55
  Bottom 0.254: U401.38 140.42,113.65 v140.74,113.32 | v154.41,111.55 R413.2
SCL@U5  (via drill 0.5)
  Top 0.254: v140.74,51.22 144.88,51.22 145.65,50.46 153.39,50.46 v154.28,49.57
  Bottom 0.254: U501.38 140.31,51.65 v140.74,51.22 | v154.28,49.57 R513.2
SDA@U1  (via drill 0.5)
  Top 0.254: v141.25,300.27 144.63,300.27 146.03,298.87 151.36,298.87 v151.72,299.23
  Bottom 0.254: U101.39 141.08,300.15 v141.25,300.27 | v151.72,299.23 R112.2
SDA@U2  (via drill 0.5)
  Top 0.254: v141.28,238.14 144.65,238.14 145.9,236.9 v154.41,236.9
  Bottom 0.254: U201.39 141.22,238.15 v141.28,238.14 | v154.41,236.9 154.79,237.28 R212.2
SDA@U3  (via drill 0.5)
  Top 0.254: v141.25,176.14 144.68,176.14 145.9,174.92 v154.26,174.92
  Bottom 0.254: U301.39 141.19,176.15 v141.25,176.14 | v154.26,174.92 154.87,175.53 R312.2
SDA@U4  (via drill 0.5)
  Top 0.254: v141.3,114.16 144.68,114.16 145.9,112.94 v154.41,112.94
  Bottom 0.254: U401.39 141.2,114.15 v141.3,114.16 | R412.2 155.55,113.58 155.17,113.2 154.66,113.2 v154.41,112.94
SDA@U5  (via drill 0.5)
  Top 0.254: v141.28,52.16 144.71,52.16 145.9,50.97 153.65,50.97 v154.28,51.6
  Bottom 0.254: U501.39 141.19,52.15 v141.28,52.16 | v154.28,51.6 R512.2
TXD  (via drill 0.5)
  Top 0.254: v237.85,50.97 230.64,50.97 226.07,46.39 220.45,46.39 220.32,46.52 219.69,46.52 219.08,45.92 v219.08,45.07
  Bottom 0.254: v237.85,50.97 250.37,50.97 259.18,42.16 259.18,22.01 263.75,17.44 263.75,13.12 261.34,10.71 J604.5 | v219.08,45.07 219.08,44.18 U704.48
V+  (via drill 0.5)
  Top 0.406: U601.7 276.71,7.66 275.69,6.64 R602.1 C601.1
  Top 0.61: R111.1 298.35,324.35 297.54,325.16 270.11,325.16 | 242.29,325.16 270.11,325.16 | 214.1,325.16 242.29,325.16 | 186.03,325.16 214.1,325.16 | R110.1 270.25,325.01 270.11,325.16 | R109.1 242.15,325.02 242.29,325.16 | R108.1 214.05,325.11 214.1,325.16 | R107.1 185.95,325.08 186.03,325.16 | R101.1 18.61,325.16 45.57,325.16 | 73.64,325.16 45.57,325.16 | 101.7,325.16 73.64,325.16 | 129.77,325.16 101.7,325.16 | 157.96,325.16 163.42,325.16 C101.1 166.59,324 v166.6,324.02 v167.62,324.02 v168.63,324.02 | 157.96,325.16 129.77,325.16 | 186.03,325.16 178.62,325.16 C102.1 175.5,324 v175.49,324.02 v174.47,324.02 v173.46,324.02 | R105.1 129.75,325.14 129.77,325.16 | R104.1 101.65,325.11 101.7,325.16 | R103.1 73.55,325.07 73.64,325.16 | R102.1 45.45,325.04 45.57,325.16 | R114.2 17.02,277.53 43.79,277.53 | 71.86,277.53 43.79,277.53 | 100.18,277.53 71.86,277.53 | 128.12,277.53 100.18,277.53 | 156.19,277.53 164.01,277.53 C105.1 164.52,278.04 v166.6,278.04 v167.62,278.04 v168.63,278.04 | 156.19,277.53 128.12,277.53 | R118.2 128.05,277.53 128.12,277.53 | R117.2 99.95,277.53 100.18,277.53 | R115.2 43.75,277.58 43.79,277.53 | R116.2 71.85,277.54 71.86,277.53 | 268.58,277.41 295.16,277.41 R124.2 | 240.39,277.41 268.58,277.41 | 212.45,277.41 240.39,277.41 | 184.13,277.41 212.45,277.41 | 184.13,277.41 178.28,277.41 C106.1 177.64,278.04 v175.49,278.04 v174.47,278.04 v173.46,278.04 | R123.2 268.55,277.44 268.58,277.41 | R122.2 240.45,277.47 240.39,277.41 | R121.2 212.35,277.5 212.45,277.41 | R120.2 184.25,277.53 184.13,277.41 | R211.1 298.35,262.35 297.54,263.16 270.11,263.16 | 242.29,263.16 270.11,263.16 | 214.1,263.16 242.29,263.16
  Top 0.61: 186.03,263.16 214.1,263.16 | R210.1 270.25,263.01 270.11,263.16 | R209.1 242.15,263.02 242.29,263.16 | R208.1 214.05,263.11 214.1,263.16 | R207.1 185.95,263.08 186.03,263.16 | R201.1 18.61,263.16 45.57,263.16 | 73.64,263.16 45.57,263.16 | 101.7,263.16 73.64,263.16 | 129.77,263.16 101.7,263.16 | 157.84,263.16 129.77,263.16 | 157.84,263.16 163.42,263.16 C201.1 166.59,262 v166.6,262.02 v167.62,262.02 v168.63,262.02 | 186.03,263.16 178.62,263.16 C202.1 175.5,262 v175.49,262.02 v174.47,262.02 v173.46,262.02 | R205.1 129.75,263.14 129.77,263.16 | R204.1 101.65,263.11 101.7,263.16 | R203.1 73.55,263.07 73.64,263.16 | R202.1 45.45,263.04 45.57,263.16 | R214.2 17.02,215.53 43.79,215.53 | 71.86,215.53 43.79,215.53 | 100.18,215.53 71.86,215.53 | 128.12,215.53 100.18,215.53 | 156.19,215.53 128.12,215.53 | 156.19,215.53 164.01,215.53 C205.1 164.52,216.04 v166.6,216.04 v167.62,216.04 v168.63,216.04 | R218.2 128.05,215.53 128.12,215.53 | R217.2 99.95,215.53 100.18,215.53 | R215.2 43.75,215.58 43.79,215.53 | R216.2 71.85,215.54 71.86,215.53 | 268.58,215.41 295.16,215.41 R224.2 | 240.39,215.41 268.58,215.41 | 212.45,215.41 240.39,215.41 | 184.13,215.41 212.45,215.41 | 184.13,215.41 178.28,215.41 C206.1 177.64,216.04 v175.49,216.04 v174.47,216.04 v173.46,216.04 | R223.2 268.55,215.44 268.58,215.41 | R222.2 240.45,215.47 240.39,215.41 | R221.2 212.35,215.5 212.45,215.41 | R220.2 184.25,215.53 184.13,215.41 | R311.1 298.35,200.35 297.54,201.16 270.11,201.16 | 242.29,201.16 270.11,201.16 | 214.1,201.16 242.29,201.16 | 186.03,201.16 214.1,201.16 | R310.1 270.25,201.02 270.11,201.16 | R309.1 242.15,201.02 242.29,201.16
  Top 0.61: R308.1 214.05,201.11 214.1,201.16 | R307.1 185.95,201.08 186.03,201.16 | R301.1 18.61,201.16 45.57,201.16 | 73.64,201.16 45.57,201.16 | 101.7,201.16 73.64,201.16 | 129.77,201.16 101.7,201.16 | 157.84,201.16 129.77,201.16 | 157.84,201.16 163.42,201.16 C301.1 166.59,200 v166.6,200.02 v167.62,200.02 v168.63,200.02 | 186.03,201.16 178.49,201.16 C302.1 175.38,200 v175.36,200.02 v174.35,200.02 v173.33,200.02 | R305.1 129.75,201.14 129.77,201.16 | R304.1 101.65,201.11 101.7,201.16 | R303.1 73.55,201.07 73.64,201.16 | R302.1 45.45,201.04 45.57,201.16 | R314.2 17.02,153.53 43.79,153.53 | 71.86,153.53 43.79,153.53 | 100.18,153.53 71.86,153.53 | 128.12,153.53 100.18,153.53 | 156.06,153.53 128.12,153.53 | 156.06,153.53 164.01,153.53 C305.1 164.52,154.04 v166.6,154.04 v167.62,154.04 v168.63,154.04 | R318.2 128.05,153.53 128.12,153.53 | R317.2 99.95,153.53 100.18,153.53 | R315.2 43.75,153.58 43.79,153.53 | R316.2 71.85,153.54 71.86,153.53 | 268.58,153.41 295.16,153.41 R324.2 | 240.39,153.41 268.58,153.41 | 212.45,153.41 240.39,153.41 | 184.13,153.41 212.45,153.41 | 184.13,153.41 178.28,153.41 C306.1 177.64,154.04 v175.49,154.04 v174.47,154.04 v173.46,154.04 | R323.2 268.55,153.44 268.58,153.41 | R322.2 240.45,153.47 240.39,153.41 | R321.2 212.35,153.5 212.45,153.41 | R320.2 184.25,153.53 184.13,153.41 | R411.1 298.35,138.35 297.54,139.16 270.11,139.16 | 242.29,139.16 270.11,139.16 | 214.1,139.16 242.29,139.16 | 186.03,139.16 214.1,139.16 | R410.1 270.25,139.01 270.11,139.16 | R409.1 242.15,139.02 242.29,139.16 | R408.1 214.05,139.11 214.1,139.16 | R407.1 185.95,139.08 186.03,139.16 | R401.1 18.61,139.16 45.57,139.16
